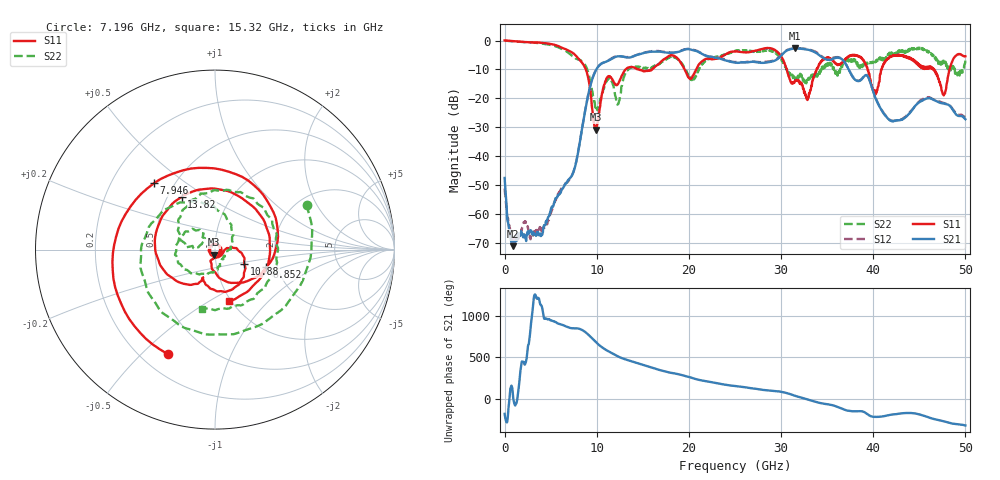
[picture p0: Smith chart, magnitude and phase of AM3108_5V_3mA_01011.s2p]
# Hz S DB R 50.0
!freq dBS11 angS11 dBS21 angS21 dBS12 angS12 dBS22 angS22
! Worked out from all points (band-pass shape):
!   1601 points, 10 MHz to 50 GHz, reference 50 ohm
!   highest |S21| = -2.72 dB at 31.53 GHz (marker M1); lowest = -71.3 dB at 947.3 MHz (marker M2)
!   |S21| within 3 dB of the highest: 13.79 GHz to 22.6 GHz (8.806 GHz wide, 48.4 % of centre); 29.87 GHz to 34.44 GHz (4.569 GHz wide, 14.2 % of centre)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
!   lowest |S11| = -30.9 dB at 9.883 GHz (marker M3), VSWR 1.06, Z = 49.1 - j2.7 ohm
!   |S11| at or under -10 dB: 8.818 GHz to 13.13 GHz (4.31 GHz wide, 39.3 % of centre); 30.62 GHz to 33.85 GHz (3.229 GHz wide, 10 % of centre); 46.62 GHz to 48.29 GHz (1.665 GHz wide, 3.51 % of centre)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
!   |S22| runs from -24.1 to 0.0 dB; largest |S21 - S12| = 0.026
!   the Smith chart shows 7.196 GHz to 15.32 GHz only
!   S11 on the Smith chart (normalised r, x): 7.196 GHz: 0.31, -0.60; 7.946 GHz: 0.39, +0.38; 8.852 GHz: 1.75, -0.37; 10.88 GHz: 1.37, -0.23; 13.82 GHz: 0.59, +0.39; 15.32 GHz: 0.97, -0.61
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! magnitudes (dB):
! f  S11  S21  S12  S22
! 10 MHz  0.0  -47.6  -51.3  0.0
! 947.3 MHz  -0.2  -71.3  -69.1  -0.3
! 3.915 GHz  -0.8  -67.0  -65.5  -1.0
! 7.196 GHz  -3.9  -47.4  -47.4  -4.9
! 7.946 GHz  -6.0  -39.4  -39.2  -6.5
! 8.352 GHz  -7.4  -31.7  -31.6  -7.1
! 8.852 GHz  -10.4  -22.5  -22.4  -9.0
! 9.883 GHz  -30.9  -10.5  -10.4  -23.0
! 10.88 GHz  -14.8  -7.5  -7.4  -15.6
! 12.32 GHz  -15.1  -5.5  -5.4  -22.0
! 13.82 GHz  -9.2  -5.7  -5.5  -9.3
! 15.32 GHz  -10.5  -4.2  -4.0  -9.4
! 16.69 GHz  -8.2  -3.8  -3.6  -8.4
! 25 GHz  -3.7  -7.7  -7.4  -3.7
! 29.16 GHz  -3.0  -7.1  -7.0  -3.7
! 31.53 GHz  -14.0  -2.7  -2.6  -13.7
! 33.35 GHz  -15.4  -3.5  -3.4  -12.7
! 38 GHz  -5.0  -13.5  -13.4  -6.6
! 40.22 GHz  -18.8  -19.7  -19.5  -7.6
! 41.69 GHz  -6.0  -27.3  -27.2  -5.1
! 47.66 GHz  -19.0  -21.9  -21.7  -7.7
! 50 GHz  -5.5  -27.3  -26.5  -6.9
